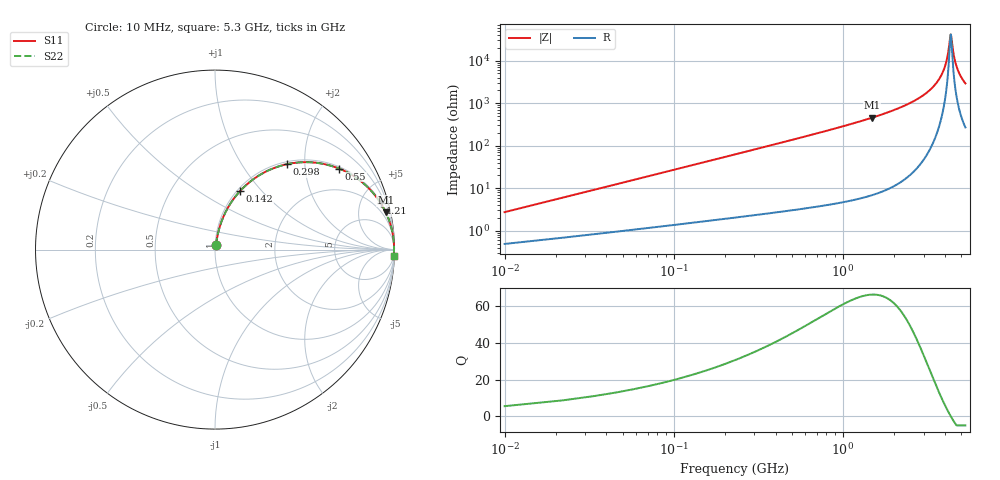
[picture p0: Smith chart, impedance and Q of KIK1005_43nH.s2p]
!version-3
!date-01.2023
!Series
# MHz S RI R 50
!Freq ReS11 ImS11 ReS21 ImS21 ReS12 ImS12 ReS22 ImS22
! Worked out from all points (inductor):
!   442 points, 10 MHz to 5.3 GHz, reference 50 ohm
!   read as one part in series: L = 43 nH near 34 MHz
!   highest Q = 66.2 at 1.486 GHz (marker M1), where L = 48.7 nH
!   self-resonance near 4.342 GHz
!   S11 on the Smith chart (normalised r, x): 10 MHz: 1.01, +0.05; 142 MHz: 1.03, +0.77; 298 MHz: 1.05, +1.62; 550 MHz: 1.06, +3.02; 1.21 GHz: 1.11, +7.09; 5.3 GHz: 6, -58
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10  0.00561 0.0267  0.9944 -0.0267  0.9944 -0.0267  0.00561 0.0267
46  0.0243 0.1201  0.9757 -0.1201  0.9757 -0.1201  0.0243 0.1201
70  0.0449 0.1786  0.9551 -0.1786  0.9551 -0.1786  0.0449 0.1786
142  0.1389 0.3254  0.8611 -0.3254  0.8611 -0.3254  0.1389 0.3254
298  0.3986 0.4755  0.6014 -0.4755  0.6014 -0.4755  0.3986 0.4755
550  0.6915 0.4514  0.3085 -0.4514  0.3085 -0.4514  0.6915 0.4514
898  0.8611 0.3374  0.1389 -0.3374  0.1389 -0.3374  0.8611 0.3374
1210  0.9228 0.2592  0.0772 -0.2592  0.0772 -0.2592  0.9228 0.2592
1486  0.951 0.2084  0.049 -0.2084  0.049 -0.2084  0.951 0.2084
1774  0.9682 0.1678  0.0318 -0.1678  0.0318 -0.1678  0.9682 0.1678
2662  0.9906 0.0858  0.00939 -0.0858  0.00939 -0.0858  0.9906 0.0858
3538  0.9967 0.035  0.00326 -0.035  0.00326 -0.035  0.9967 0.035
3826  0.9974 0.0215  0.00261 -0.0215  0.00261 -0.0215  0.9974 0.0215
4042  0.9976 0.0122  0.0024 -0.0122  0.0024 -0.0122  0.9976 0.0122
4174  0.9976 0.00673  0.00237 -0.00673  0.00237 -0.00673  0.9976 0.00673
4330  0.9976 0.000501  0.00242 -0.000501  0.00242 -0.000501  0.9976 0.000501
4366  0.9976 -0.000903  0.00244 0.000903  0.00244 0.000903  0.9976 -0.000903
4426  0.9975 -0.00322  0.00249 0.00322  0.00249 0.00322  0.9975 -0.00322
4558  0.9974 -0.0082  0.00263 0.0082  0.00263 0.0082  0.9974 -0.0082
4726  0.9971 -0.0143  0.00289 0.0143  0.00289 0.0143  0.9971 -0.0143
4978  0.9966 -0.0232  0.00342 0.0232  0.00342 0.0232  0.9966 -0.0232
5300  0.9957 -0.0339  0.00431 0.0339  0.00431 0.0339  0.9957 -0.0339
